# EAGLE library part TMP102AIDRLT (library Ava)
Temperature Sensor
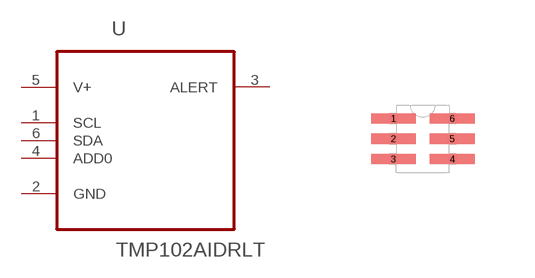
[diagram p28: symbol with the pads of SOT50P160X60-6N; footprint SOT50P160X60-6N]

Designator prefix U

## TMP102AIDRLT (MPN: TMP102AIDRLT; OC_FARNELL: 1652477; OC_NEWARK: 53M3987; PACKAGE: SOT-23-6; SUPPLIER: Texas Instruments)  [SOT50P160X60-6N]
1  SCL
2  GND  pas
3  ALERT  out
4  ADD0  in
5  V+  pwr
6  SDA

## Footprint SOT50P160X60-6N (pad centres in mm)
smd 1.118 x 0.254: 1 -0.737,0.508; 2 -0.737,0; 3 -0.737,-0.508; 4 0.737,-0.508; 5 0.737,0; 6 0.737,0.508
